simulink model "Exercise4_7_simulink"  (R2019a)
settings: Solver=ode4  StartTime=0.0  StopTime=6.0  FixedStep=deltat  RelTol=1e-3  EnableMultiTasking=on
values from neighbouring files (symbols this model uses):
  alpha = [a11    0   a12     0    [Exercise4_5.m]    (also in Exercise4_7.m = 30; Exercise2_12.m = a*((3*a)+(2*b))/(6*E*I); Exercise2_15.m = 0; Exercise2_16.m = eval(a12))
  beta1 = 0    [Exercise4_7.m]
  beta2 = 240*pi/18    (= 41.8879020479)    [Exercise4_7.m]
  C = B*(inv(K)+inv(D))*A    [Exercise4_5.m]    (also in Exercise4_7.m = [cxx(i) cxy(i) 0 0; cyx(i) cyy(i) 0 0; 0 0 cxx(i) cxy(i); 0 ; Exercise3_3.m = C + (g + xmax2 * cos(xi(j))).^(n-1) * sin(xi(j)) * cos(xi(j); Exercise3_3_general_ball.m = C + (g(i) + xmax2 * cos(xi(j)))^(n-1) * sin(xi(j)) * cos(xi(; Exercise3_3_general_roller.m = C + (g(i) + xmax2 * cos(xi(j)))^(n-1) * sin(xi(j)) * cos(xi()
  G = [0 -ip 0 ip; ip 0 -ip 0; 0 ip 0 -ip; -ip 0 ip 0]    [Exercise4_7.m]    (also in Exercise5_16.m = [0   0   0   0)
  K = [kA 0; 0 kB]    [Exercise4_1.m]    (also in Exercise4_10.m = 2*[kxx*L kxy*L;kyx*L kyy*L]; Exercise4_11.m = 0.5*L^2*[kxx kxy;kyx kyy]; Exercise4_16.m = [kxa+kxb            -(kxa*Lag - kxb*Lbg); Exercise4_19.m = [kA+kB                   -(kA*Lag + kB*Lbg))
  l1_bar = L1/L    (= 0.5)    [Exercise4_7.m]
  l2_bar = L2/L    (= 0.5)    [Exercise4_7.m]
  M1 = [ m   0    [Exercise4_20.m]    (also in Exercise4_7.m = inv(M); Exercise2_17.m = F*z/2; Exercise2_6.m = M)
  omega0 = 5    [Exercise4_7.m]
  r1_bar = R1/L    (= 0.305882352941)    [Exercise4_7.m]
  r2_bar = R2/L    (= 0.305882352941)    [Exercise4_7.m]
  u1 = m1*e1    (= 9e-05)    [Exercise4_7.m]
  u2 = m2*e2    (= 0.00025)    [Exercise4_7.m]

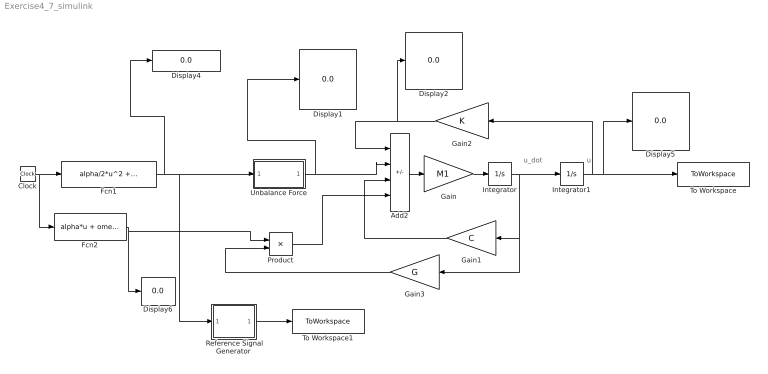
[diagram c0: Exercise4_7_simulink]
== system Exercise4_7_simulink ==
  note: u_dot
  note: u
  " Reference Signal Generator" : Subsystem
  Add2 : Sum  Inputs=-+-+  InputSameDT=on
  Clock : Clock
  Display{1..2,4..6} (5 alike) : Display
  Fcn1 : Fcn  Expr=alpha/2*u^2 + omega0*u
  Fcn2 : Fcn  Expr=alpha*u + omega0
  Gain : Gain  Gain=M1  Multiplication=Matrix(K*u)
  Gain1 : Gain  Gain=C  Multiplication=Matrix(K*u)
  Gain2 : Gain  Gain=K  Multiplication=Matrix(K*u)
  Gain3 : Gain  Gain=G  Multiplication=Matrix(K*u)
  Integrator : Integrator
  Integrator1 : Integrator
  Product : Product
  To Workspace : ToWorkspace  VariableName=Displacement  SampleTime=-1
  To Workspace1 : ToWorkspace  VariableName=Reference  SampleTime=-1
  Unbalance Force : Subsystem
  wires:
  Clock/1 -> Fcn1/1, Fcn2/1
  Gain/1 -> Integrator/1
  Integrator1/1 -> Display5/1, To Workspace/1, Gain2/1
  Integrator/1 -> Integrator1/1, Gain3/1, Gain1/1
  Add2/1 -> Gain/1
  Gain2/1 -> Display2/1, Add2/1
  Gain1/1 -> Add2/3
  Unbalance Force/1(Out1) -> Display1/1, Add2/2
  " Reference Signal Generator"/1(Out4) -> To Workspace1/1
  Fcn1/1 -> Display4/1, Unbalance Force/1(In1), " Reference Signal Generator"/1(In4)
  Fcn2/1 -> Product/1, Display6/1
  Gain3/1 -> Product/2
  Product/1 -> Add2/4

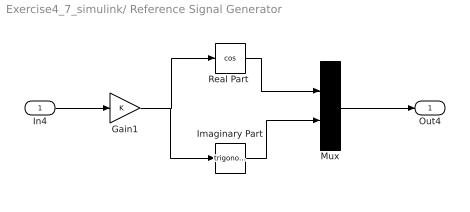
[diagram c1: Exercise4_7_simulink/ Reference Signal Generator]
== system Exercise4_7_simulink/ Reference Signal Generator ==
  In4 : Inport
  Gain1 : Gain
  Imaginary Part : Trigonometry
  Mux : Mux  Inputs=2
  "Real Part " : Trigonometry  Operator=cos
  Out4 : Outport
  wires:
  Gain1/1 -> Imaginary Part/1, "Real Part "/1
  In4/1 -> Gain1/1
  Mux/1 -> Out4/1
  "Real Part "/1 -> Mux/1
  Imaginary Part/1 -> Mux/2

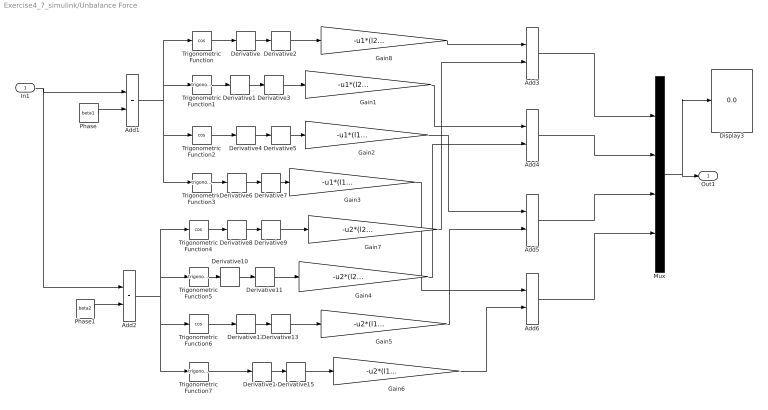
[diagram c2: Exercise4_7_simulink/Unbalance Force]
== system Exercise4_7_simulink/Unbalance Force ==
  In1 : Inport
  Add{1..6} (6 alike) : Sum  InputSameDT=on
  Derivative{,1..15} (16 alike) : Derivative
  Display3 : Display
  Gain1 : Gain  Gain=-u1*(l2_bar+r1_bar)
  Gain2 : Gain  Gain=-u1*(l1_bar-r1_bar)
  Gain3 : Gain  Gain=-u1*(l1_bar-r1_bar)
  Gain4 : Gain  Gain=-u2*(l2_bar-r2_bar)
  Gain5 : Gain  Gain=-u2*(l1_bar+r2_bar)
  Gain6 : Gain  Gain=-u2*(l1_bar+r2_bar)
  Gain7 : Gain  Gain=-u2*(l2_bar-r2_bar)
  Gain8 : Gain  Gain=-u1*(l2_bar+r1_bar)
  Mux : Mux
  Phase : Constant  Value=beta1
  Phase1 : Constant  Value=beta2
  Trigonometric Function{,2,4,6} (4 alike) : Trigonometry  Operator=cos
  Trigonometric Function{1,3,5,7} (4 alike) : Trigonometry
  Out1 : Outport
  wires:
  In1/1 -> Add2/1, Add1/1
  Trigonometric Function2/1 -> Derivative4/1
  Trigonometric Function1/1 -> Derivative1/1
  Trigonometric Function3/1 -> Derivative6/1
  Add1/1 -> Trigonometric Function/1, Trigonometric Function1/1, Trigonometric Function3/1, Trigonometric Function2/1
  Phase/1 -> Add1/2
  Trigonometric Function/1 -> Derivative/1
  Phase1/1 -> Add2/2
  Add2/1 -> Trigonometric Function4/1, Trigonometric Function5/1, Trigonometric Function7/1, Trigonometric Function6/1
  Trigonometric Function6/1 -> Derivative12/1
  Trigonometric Function7/1 -> Derivative14/1
  Trigonometric Function4/1 -> Derivative8/1
  Gain7/1 -> Add3/2
  Gain4/1 -> Add4/2
  Gain5/1 -> Add5/2
  Gain6/1 -> Add6/2
  Gain3/1 -> Add6/1
  Gain2/1 -> Add5/1
  Gain1/1 -> Add4/1
  Gain8/1 -> Add3/1
  Add6/1 -> Mux/4
  Add5/1 -> Mux/3
  Add4/1 -> Mux/2
  Add3/1 -> Mux/1
  Derivative/1 -> Derivative2/1
  Derivative2/1 -> Gain8/1
  Derivative1/1 -> Derivative3/1
  Derivative3/1 -> Gain1/1
  Derivative4/1 -> Derivative5/1
  Derivative5/1 -> Gain2/1
  Derivative6/1 -> Derivative7/1
  Derivative7/1 -> Gain3/1
  Derivative9/1 -> Gain7/1
  Derivative8/1 -> Derivative9/1
  Trigonometric Function5/1 -> Derivative10/1
  Derivative10/1 -> Derivative11/1
  Derivative11/1 -> Gain4/1
  Derivative13/1 -> Gain5/1
  Derivative12/1 -> Derivative13/1
  Derivative15/1 -> Gain6/1
  Derivative14/1 -> Derivative15/1
  Mux/1 -> Display3/1, Out1/1
